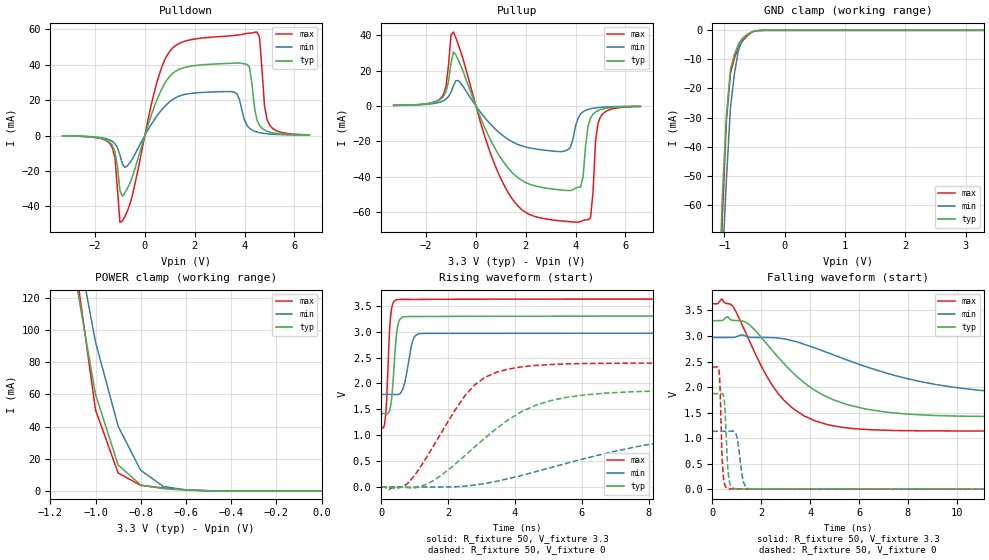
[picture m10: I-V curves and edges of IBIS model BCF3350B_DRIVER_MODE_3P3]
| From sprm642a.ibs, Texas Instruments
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|   Model Cell BCF3350B_DRIVER_MODE_3P3
|BCF3350B_DRIVER_MODE_3P3
[Model]   BCF3350B_DRIVER_MODE_3P3
Model_type   I/O
Polarity   Non-Inverting
Enable   Active-Low
Vinl =  0.8
Vinh =  2
Cref =  15.0000pF
Rref =  100.0000M
Vref =  0V
Vmeas =  1.65
C_comp   1.081689p   0.9467568p   1.2214p
[Model Spec]
Vinl   0.8   0.8   0.8
Vinh   2   2   2
[Temperature Range]   25   155   -40
[Voltage Range]   3.3   2.97   3.63
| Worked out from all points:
|   slope of the pulldown table from 0 to 0.495 V, typ, clamps not added: 24.2 ohm
|   slope of the pullup table from 0 to 0.495 V, typ, clamps not added: 29.8 ohm
|   GND clamp passes 1 mA (typ) near -0.59 V on its own axis
|   POWER clamp passes 1 mA (typ) near -0.65 V on its own axis
|   rising waveform, R_fixture 50, V_fixture 3.3: 20-80 % time 127ps typ, 199ps min, 102ps max; typ from 1.42 V to 3.3 V
|   rising waveform, R_fixture 50, V_fixture 0: 20-80 % time 2.25ns typ, 4.65ns min, 1.45ns max; typ from 0 V to 1.87 V
|   falling waveform, R_fixture 50, V_fixture 3.3: 20-80 % time 2.66ns typ, 5.11ns min, 1.86ns max; typ from 3.3 V to 1.42 V
|   falling waveform, R_fixture 50, V_fixture 0: 20-80 % time 115ps typ, 183ps min, 93.3ps max; typ from 1.87 V to 0 V
| Nom Voltages:
|   VDD=1.2, VDDS=3.3, VSS=0
| Min Voltages:
|   VDD=1.08, VDDS=2.97, VSS=0
| Max Voltages:
|   VDD=1.32, VDDS=3.63, VSS=0
[POWER_clamp]
|   voltage   I(typ)   I(min)   I(max)
-3.3V     2.318A     2.595A     3.049A
-1.1V     141.5mA    168mA      152.3mA
-1.067V   114.3mA    142.9mA    118.3mA
-1.033V   87.17mA    117.8mA    84.37mA
-1V       60.01mA    92.63mA    50.4mA
-900mV    16.17mA    40.25mA    11.16mA
-800mV    3.655mA    12.81mA    3.461mA
-700mV    1.415mA    2.754mA    1.844mA
-600mV    504.3uA    641.1uA    658.2uA
-500mV    86.55uA    148.2uA    94.22uA
0V        39.59pA    2.724nA    9.668pA
[Pulldown]
|   voltage   I(typ)   I(min)   I(max)
-3.3V     -252.1uA   -234.7uA   -277.7uA
-1.4V     -3.919mA   -2.547mA   -4.608mA
-1.2V     -9.103mA   -4.609mA   -12.64mA
-900mV    -34.3mA    -16.21mA   -48.36mA
1V        33.43mA    19.12mA    47.58mA
3.6V      40.87mA    24.35mA    56.5mA
4.1V      40.18mA    5.681mA    57.63mA
4.5V      8.744mA    1.956mA    58.39mA
4.6V      5.703mA    1.616mA    55.56mA
4.8V      3.099mA    1.152mA    16.91mA
5V        1.969mA    859.8uA    6.049mA
6.6V      281.1uA    214.2uA    387.2uA
[Pullup]
|   voltage   I(typ)   I(min)   I(max)
-3.3V     278.9uA    242.8uA    252.3uA
-1.4V     3.885mA    2.29mA     4.485mA
-900mV    30.46mA    11.45mA    41.76mA
500mV     -16.76mA   -9.024mA   -23.45mA
1.4V      -36.9mA    -19.86mA   -51.44mA
3.6V      -47.86mA   -25.33mA   -65.39mA
4.1V      -46.11mA   -6.928mA   -65.87mA
4.3V      -40.29mA   -3.368mA   -64.88mA
4.6V      -6.878mA   -1.656mA   -63.29mA
4.8V      -3.477mA   -1.154mA   -20.01mA
5V        -2.143mA   -846.4uA   -6.19mA
6.6V      -290.9uA   -205.6uA   -395.4uA
[GND_clamp]
|   voltage   I(typ)   I(min)   I(max)
-3.3V     -1.888A    -1.585A    -3.154A
-1.1V     -95.78mA   -113.9mA   -112.1mA
-1.033V   -56.7mA    -80.3mA    -63.61mA
-966.7mV  -29.24mA   -51.23mA   -31.16mA
-900mV    -13.41mA   -26.67mA   -14.73mA
-833.3mV  -8.233mA   -14.78mA   -9.457mA
-766.7mV  -4.676mA   -6.859mA   -5.761mA
-700mV    -2.737mA   -2.908mA   -3.644mA
-566.7mV  -742.7uA   -781uA     -966.3uA
-500mV    -188.9uA   -280.3uA   -215.5uA
-366.7mV  -8.774uA   -27.7uA    -8.181uA
3.3V      39.59pA    4.205uA    5.4pA
[Ramp]
| variable   typ   min   max
dV/dt_f   1.175455/2.6995308n 0.73863336/5.194549n   1.5502169/1.891376n
dV/dt_r  1.1439003/2.2847426n 0.69345692/4.7193079n   1.462025/1.4734427n
R_load = 50
[Rising Waveform]
R_fixture = 50
V_fixture = 3.3
V_fixture_min = 2.97
V_fixture_max = 3.63
|   time   V(typ)   V(min)   V(max)
0s        1.419V     1.788V     1.14V
82.8ps    1.418V     1.788V     1.173V
135.5ps   1.416V     1.788V     1.437V
269.6ps   1.529V     1.788V     3.24V
343.1ps   1.966V     1.787V     3.538V
456ps     2.961V     1.784V     3.617V
598.6ps   3.268V     1.837V     3.623V
930.1ps   3.293V     2.806V     3.623V
1.163ns   3.293V     2.962V     3.622V
20.01ns   3.3V       2.97V      3.63V
[Rising Waveform]
R_fixture = 50
V_fixture = 0
V_fixture_min = 0
V_fixture_max = 0
|   time   V(typ)   V(min)   V(max)
0s        0V         0V         0V
766.6ps   -4.653mV   -13.13mV   53.5mV
1.376ns   56.95mV    -2.28mV    592.3mV
2.196ns   432mV      0V         1.473V
2.794ns   771.2mV    35.65mV    1.97V
3.813ns   1.301V     160.8mV    2.279V
4.625ns   1.578V     294mV      2.347V
6.034ns   1.773V     538.8mV    2.383V
10.55ns   1.868V     1.017V     2.392V
20.06ns   1.87V      1.132V     2.392V
[Falling Waveform]
R_fixture = 50
V_fixture = 3.3
V_fixture_min = 2.97
V_fixture_max = 3.63
|   time   V(typ)   V(min)   V(max)
0s        3.3V       2.97V      3.63V
382.8ps   3.301V     2.97V      3.723V
874.8ps   3.304V     2.972V     3.555V
1.542ns   3.211V     2.975V     2.872V
2.287ns   2.81V      2.97V      2.16V
2.93ns    2.457V     2.943V     1.74V
4.747ns   1.795V     2.667V     1.259V
7.128ns   1.507V     2.271V     1.153V
9.901ns   1.433V     1.994V     1.14V
20.01ns   1.419V     1.788V     1.14V
[Falling Waveform]
R_fixture = 50
V_fixture = 0
V_fixture_min = 0
V_fixture_max = 0
|   time   V(typ)   V(min)   V(max)
0s        1.87V      1.132V     2.392V
281.1ps   1.871V     1.132V     2.287V
402.9ps   1.871V     1.132V     576.6mV
456.7ps   1.827V     1.132V     215.2mV
626.5ps   452.3mV    1.132V     11.85mV
730.5ps   89.53mV    1.136V     4.605mV
960.1ps   8.893mV    1.089V     3.962mV
1.279ns   5.244mV    127.4mV    3.922mV
1.55ns    4.559mV    6.922mV    2.199mV
20.06ns   0V         0V         0V
